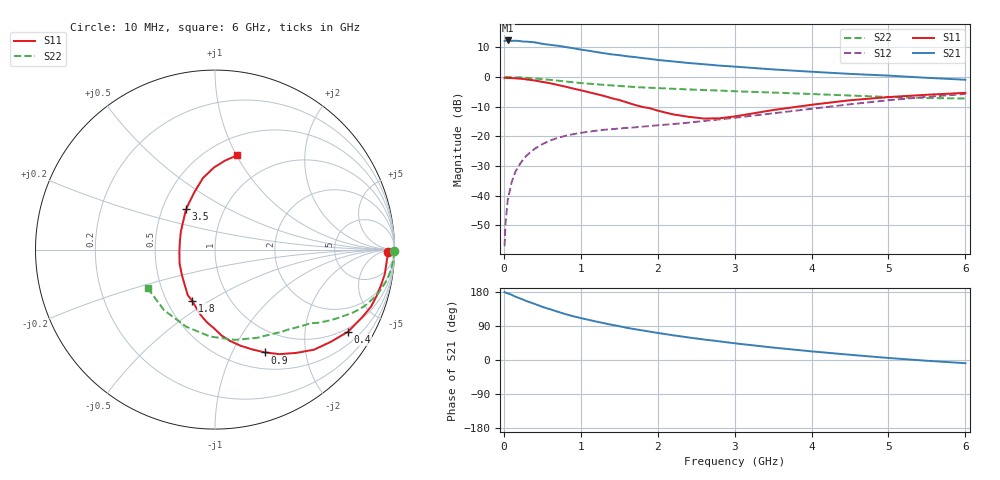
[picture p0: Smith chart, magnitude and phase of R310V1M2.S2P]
! SIEMENS Small Signal Semiconductors
! BFR181
! Si NPN RF Bipolar Junction Transistor in SOT23
! VCE = 10 V  IC = 1.2 mA
! Common Emitter S-Parameters:  May  1996
# GHz  S  MA  R  50
!  f  S11  S21  S12  S22
! GHz  MAG  ANG  MAG  ANG  MAG  ANG  MAG  ANG
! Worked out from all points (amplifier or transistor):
!   36 points, 10 MHz to 6 GHz, reference 50 ohm
!   highest |S21| = 12.3 dB at 50 MHz (marker M1)
!   |S21| within 3 dB of that: start of sweep to 985.4 MHz
!   unconditionally stable (mu >= 1): 1.982 GHz to 3.667 GHz
!   at 250 MHz: K = 0.17, MSG = 19.9 dB, |S12| = -27.9 dB
!   at 1.4 GHz: K = 0.80, MSG = 12.6 dB, |S12| = -17.6 dB
!   at 6 GHz: K = 0.87, MSG = 2.4 dB, |S12| = -5.8 dB
!   S11 on the Smith chart (normalised r, x): 10 MHz: 44, -18; 400 MHz: 0.87, -3.31; 900 MHz: 0.70, -1.35; 1.8 GHz: 0.67, -0.42; 3.5 GHz: 0.66, +0.32; 6 GHz: 0.68, +1.00
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0.01  0.9617 -0.9  4.033 179.2  0.0014 76.4  0.9977 -0.4
0.02  0.9626 -1.8  4.06 178.0  0.0032 86.1  0.9948 -0.8
0.05  0.9587 -4.2  4.118 175.9  0.0083 88.0  0.9964 -2.0
0.1  0.9558 -8.2  4.042 172.1  0.0165 85.2  0.9936 -3.9
0.15  0.9467 -11.9  4.08 167.2  0.0252 81.3  0.9875 -5.9
0.3  0.9045 -24.3  3.928 155.1  0.0478 74.9  0.9649 -11.3
0.4  0.871 -31.7  3.833 148.1  0.0614 69.9  0.9429 -14.8
0.5  0.8245 -38.6  3.614 140.3  0.0733 66.1  0.9167 -17.8
0.7  0.7316 -51.9  3.355 127.5  0.0936 59.6  0.8647 -22.9
0.9  0.6377 -64.0  3.049 115.5  0.1082 54.3  0.8117 -26.9
1.1  0.5537 -75.2  2.765 106.1  0.1191 50.9  0.7695 -30.2
1.2  0.5153 -80.7  2.634 101.4  0.1238 49.4  0.7511 -31.7
1.4  0.4379 -90.8  2.401 93.0  0.1312 47.8  0.7188 -34.2
1.6  0.3715 -102.7  2.229 84.9  0.1384 47.1  0.6913 -36.3
1.8  0.3119 -114.1  2.078 78.1  0.1451 47.5  0.6653 -38.4
2.2  0.2333 -142.1  1.824 65.2  0.1602 48.4  0.6305 -43.2
2.6  0.1986 -177.1  1.638 54.1  0.1806 50.2  0.5996 -48.3
2.8  0.2003 168.0  1.551 49.3  0.1918 50.8  0.5889 -51.3
3.5  0.2765 125.8  1.338 32.8  0.2432 51.4  0.5447 -64.5
4.5  0.4042 99.6  1.125 13.8  0.3456 46.5  0.4852 -93.1
5.5  0.5001 83.4  0.966 -2.0  0.4612 34.9  0.4409 -130.1
6  0.5383 76.9  0.896 -8.4  0.5153 27.4  0.4322 -150.2
